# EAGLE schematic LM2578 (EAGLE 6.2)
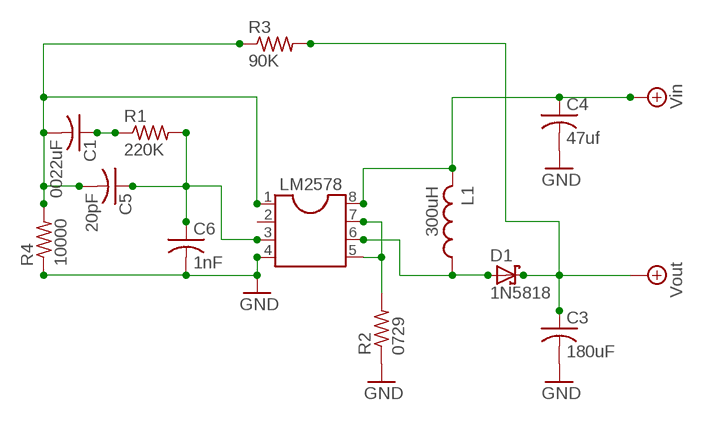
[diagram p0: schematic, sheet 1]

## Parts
C1  0022uF  C-US050-025X075  [C050-025X075]
C3  180uF  C-US050-025X075  [C050-025X075]
C4  47uf  C-US050-025X075  [C050-025X075]
C5  20pF  C-US050-025X075  [C050-025X075]
C6  1nF  C-US050-025X075  [C050-025X075]
D1  1N5818  1N5908  [C4111-15]
L1  300uH  L-USL1812  [L1812]
LM2578  DIL8  [DIL08]
R1  220K  R-US_0414/15  [0414/15]
R2  0729  R-US_0414/15  [0414/15]
R3  90K  R-US_0414/15  [0414/15]
R4  10000  R-US_0414/15  [0414/15]

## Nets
+7V: C3.1 D1.C R3.2 ; supply symbol labelled Vout
GND: C3.2 C4.2 LM2578.4 R2.1
N$1: C1.1 R1.1
N$2: C5.1 C6.1 LM2578.3 R1.2
N$3: C1.2 C5.2 LM2578.1 R3.1 R4.2
N$4: C6.2 R4.1
N$5: LM2578.5 LM2578.7 R2.2
N$8: C4.1 L1.2 LM2578.8 ; supply symbol labelled Vin
N$10: D1.A L1.1 LM2578.6
Unconnected: LM2578.2

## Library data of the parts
C1 C3-C6 = resistor:C-US: CAPACITOR, American symbol
D1 = diode:1N5908: DIODE
L1 = resistor:L-US: INDUCTOR, American symbol
LM2578 = ic-package:DIL8: Dual In Line / Socket
R1-R4 = resistor:R-US_: RESISTOR, American symbol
